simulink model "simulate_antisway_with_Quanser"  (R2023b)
settings: Solver=daessc  StartTime=0.0  StopTime=sim_stop_time  RelTol=1e-3
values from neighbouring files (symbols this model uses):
  antisway_Volt_Limit = 20.0
                
                    
                        1
                        Auto
                        
                        
                        -1.0
                        0
                        Simulink
                        Parameter
                        Default    [antisway_with_Quanser.sldd]
  dphi_gain = 0.0    [antisway_with_Quanser.sldd]
  dphi_init = 0.0    [antisway_with_Quanser.sldd]
  dtheta_gain = 0.0    [antisway_with_Quanser.sldd]
  dtheta_init = 0.0    [antisway_with_Quanser.sldd]
  phi_gain = 0.0    [antisway_with_Quanser.sldd]
  phi_init = 0.0    [antisway_with_Quanser.sldd]
  sim_stop_time = 30.0
                
                    
                        1
                        Auto
                        
                        
                        -1.0
                        0
                        Simulink
                        Parameter
                        Default    [run_FRE_data.sldd]
  theta_gain = 0.0    [antisway_with_Quanser.sldd]
  theta_init = 0.0    [antisway_with_Quanser.sldd]
libraries: checkpacklib x3, pendulumLib x1, SignalEditorBlockLib x1

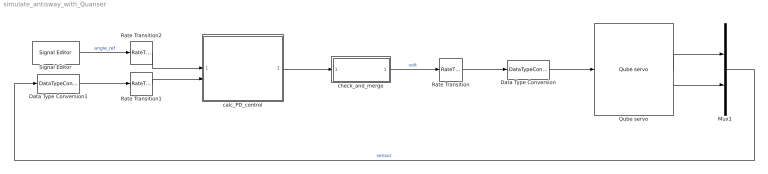
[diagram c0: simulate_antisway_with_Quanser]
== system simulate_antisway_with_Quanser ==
  Data Type Conversion : DataTypeConversion  OutDataTypeStr=double
  Data Type Conversion1 : DataTypeConversion  OutDataTypeStr=single
  Mux1 : Mux  Inputs=2
  Qube servo : pendulumLib/Qube servo  a0=[theta_init, phi_init]  w0=[dtheta_init, dphi_init]  R_m=R_m  L_m=L_m  mu_m=mu_m  K_b=K_b  n=n  rod_mass=m_r  rod_length=L_r  rod_rad=rod_rad  p_mass=m_p  p_length=L_p  p_rad=p_rad  D_r=D_r  D_p=D_p
  Rate Transition : RateTransition
  Rate Transition1 : RateTransition  OutPortSampleTime=FRE_time_step
  Rate Transition2 : RateTransition  OutPortSampleTime=FRE_time_step
  Signal Editor : SignalEditorBlockLib/Signal Editor  FileName=pendulum_reference_data.mat  ActiveScenario=Step_sequence  ActiveSignal=angle_ref  IsBus=off  OutputBusObjectStr=Bus: BusObject  SampleTime=0  Interpolate=off  ZeroCross=off  OutputAfterFinalValue=Holding final value  Unit=inherit  PreserveSignalName=on  ApplySigPropsToAllScenarios=on  ApplySigPropsToAllSignals=on
  calc_PD_control : Subsystem  ReferencedSubsystem=calc_PD_control
  check_and_merge : Subsystem
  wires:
  Qube servo/2 -> Mux1/2
  Qube servo/1 -> Mux1/1
  Rate Transition/1 -> Data Type Conversion/1
  Data Type Conversion/1 -> Qube servo/1
  Mux1/1 -> Data Type Conversion1/1  "sensor"
  Data Type Conversion1/1 -> Rate Transition1/1
  Signal Editor/1 -> Rate Transition2/1  "angle_ref"
  Rate Transition1/1 -> calc_PD_control/2
  Rate Transition2/1 -> calc_PD_control/1
  calc_PD_control/1 -> check_and_merge/1(dif_vec)
  check_and_merge/1(volt) -> Rate Transition/1  "volt"

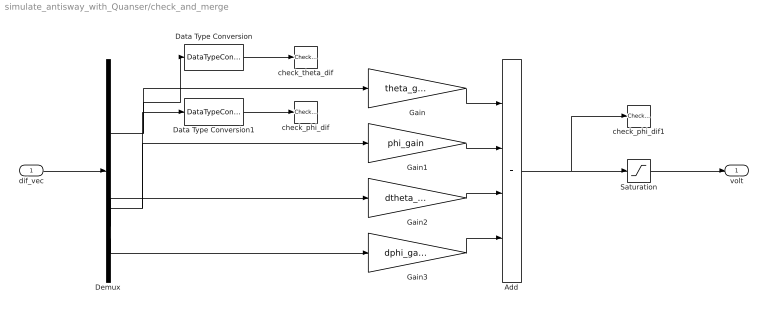
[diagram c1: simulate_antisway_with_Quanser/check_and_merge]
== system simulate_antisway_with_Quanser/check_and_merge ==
  dif_vec : Inport
  Add : Sum  Inputs=++++
  Data Type Conversion : DataTypeConversion  OutDataTypeStr=double
  Data Type Conversion1 : DataTypeConversion  OutDataTypeStr=double
  Demux : Demux
  Gain : Gain  Gain=theta_gain
  Gain1 : Gain  Gain=phi_gain
  Gain2 : Gain  Gain=dtheta_gain
  Gain3 : Gain  Gain=dphi_gain
  Saturation : Saturate  UpperLimit=antisway_Volt_Limit  LowerLimit=-antisway_Volt_Limit
  check_phi_dif : checkpacklib/Check Custom Bounds  InstantiateOnLoad=on  enabled=off  stopWhenAssertionFail=off  export=off  ViewDlgPos=[100 200 510 390]  OpenViewOnLoad=off  LaunchViewOnOpen=off  TimeUnits=seconds  EnableUpperBound=on  UpperBoundTimes=bound_info.upper_time  UpperBoundAmplitudes=bound_info.upper_value  EnableLowerBound=on  LowerBoundTimes=bound_info.lower_time  LowerBoundAmplitudes=bound_info.lower_value
  check_phi_dif1 : checkpacklib/Check Custom Bounds  InstantiateOnLoad=on  enabled=off  stopWhenAssertionFail=off  export=off  ViewDlgPos=[100 200 510 390]  OpenViewOnLoad=off  LaunchViewOnOpen=off  TimeUnits=seconds  EnableUpperBound=on  UpperBoundTimes=[0, sim_stop_time]  UpperBoundAmplitudes=[antisway_Volt_Limit, antisway_Volt_Limit]  EnableLowerBound=on  LowerBoundTimes=[0, sim_stop_time]  LowerBoundAmplitudes=[-antisway_Volt_Limit, -antisway_Volt_Limit]
  check_theta_dif : checkpacklib/Check Against Reference  InstantiateOnLoad=on  enabled=off  stopWhenAssertionFail=off  export=off  ViewDlgPos=[]  OpenViewOnLoad=off  LaunchViewOnOpen=off  TimeUnits=seconds  EnableReferenceBound=on  AbsTolerance=eps^(1/3)  RelTolerance=0.01  ReferenceTimes=[0, sim_stop_time]  ReferenceAmplitudes=[0; 0]
  volt : Outport
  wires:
  Demux/1 -> Data Type Conversion/1, Gain/1
  Demux/2 -> Gain1/1, Data Type Conversion1/1
  Demux/3 -> Gain2/1
  Demux/4 -> Gain3/1
  dif_vec/1 -> Demux/1
  Add/1 -> check_phi_dif1/1, Saturation/1
  Data Type Conversion/1 -> check_theta_dif/1
  Data Type Conversion1/1 -> check_phi_dif/1
  Gain/1 -> Add/1
  Gain1/1 -> Add/2
  Gain2/1 -> Add/3
  Gain3/1 -> Add/4
  Saturation/1 -> volt/1
